TYPE ST_ENC_Control_Output_Channel :
STRUCT
	{attribute 'displaymode':='bin'}
	Control							:	ST_ControlOutput_UINT_TO_BIT;// bit
	Number_of_output_events			:	USINT;
	{attribute 'displaymode':='bin'}
	Output_state					:	USINT;
	Threshold						:	ARRAY[1..8] OF UDINT;
	Duration						:	ARRAY[1..8] OF UDINT;
END_STRUCT
END_TYPE
